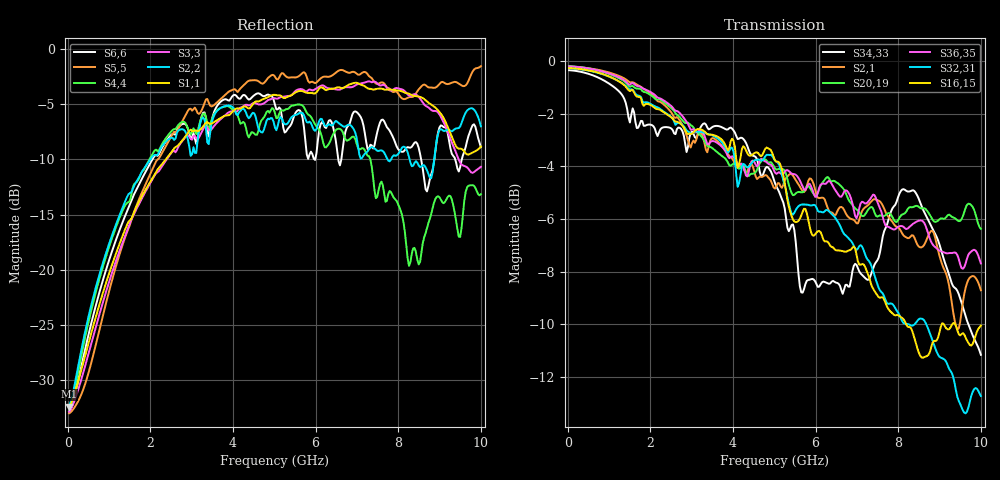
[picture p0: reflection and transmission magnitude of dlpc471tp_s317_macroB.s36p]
! Touchstone(R) file created by SIwave 2018.1.0
! Touchstone(R) file created on Tue Aug 27 06:24:33 2019
! Port[1] = DCLK_BN_DIE_161
! Port[2] = DCLK_BN_LGA_A16
! Port[3] = DCLK_BP_DIE_160
! Port[4] = DCLK_BP_LGA_A17
! Port[5] = D_BN_0__DIE_180
! Port[6] = D_BN_0__LGA_A15
! Port[7] = D_BN_1__DIE_176
! Port[8] = D_BN_1__LGA_G23
! Port[9] = D_BN_2__DIE_172
! Port[10] = D_BN_2__LGA_E23
! Port[11] = D_BN_3__DIE_166
! Port[12] = D_BN_3__LGA_A23
! Port[13] = D_BN_4__DIE_156
! Port[14] = D_BN_4__LGA_D24
! Port[15] = D_BN_5__DIE_150
! Port[16] = D_BN_5__LGA_A21
! Port[17] = D_BN_6__DIE_146
! Port[18] = D_BN_6__LGA_B25
! Port[19] = D_BN_7__DIE_142
! Port[20] = D_BN_7__LGA_A19
! Port[21] = D_BP_0__DIE_179
! Port[22] = D_BP_0__LGA_A14
! Port[23] = D_BP_1__DIE_175
! Port[24] = D_BP_1__LGA_F23
! Port[25] = D_BP_2__DIE_171
! Port[26] = D_BP_2__LGA_E24
! Port[27] = D_BP_3__DIE_165
! Port[28] = D_BP_3__LGA_A22
! Port[29] = D_BP_4__DIE_155
! Port[30] = D_BP_4__LGA_D25
! Port[31] = D_BP_5__DIE_149
! Port[32] = D_BP_5__LGA_A20
! Port[33] = D_BP_6__DIE_145
! Port[34] = D_BP_6__LGA_B24
! Port[35] = D_BP_7__DIE_141
! Port[36] = D_BP_7__LGA_A18
! S-parameters
# Hz S MA R 50.000000
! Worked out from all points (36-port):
!   299 points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, 33.44 MHz to 10 GHz, reference 50 ohm
!   strongest paths, dB at 33.44 MHz, 2.508 GHz, 5.017 GHz, 7.525 GHz, 10 GHz:
!     S16,15: -0.3, -2.1, -3.8, -9.0, -10.0
!     S32,31: -0.3, -2.1, -3.8, -8.6, -12.7
!     S36,35: -0.2, -1.7, -4.2, -5.5, -7.7
!     S20,19: -0.2, -1.8, -4.1, -5.9, -6.4
!     S2,1: -0.2, -2.0, -4.8, -5.3, -8.7
!     S34,33: -0.4, -2.6, -4.6, -7.5, -11.2
!   lowest |S11| = -32.4 dB at 33.44 MHz (marker M1), VSWR 1.05, Z = 52.4 + j0.297 ohm
!   |S11| at or under -10 dB: start of sweep to 2.371 GHz
